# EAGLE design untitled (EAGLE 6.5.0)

## Sheet 1 of 3: NAP a SERVO
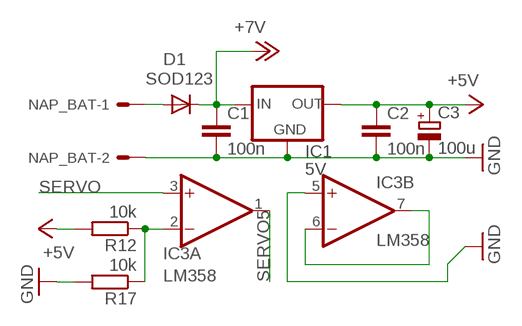
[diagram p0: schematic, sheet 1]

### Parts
C1  100n  C-EUC0805K  [C0805K]
C2  100n  C-EUC0805K  [C0805K]
C3  100u  CPOL-EUE2-5  [E2-5]
D1  SOD123  CGRM4001-G  [SOD-123_MINI-SMA]
IC1  5V  78XXL  [78XXL]
IC3  LM358  TL072D  [SO08]
NAP_BAT  22-27-2021-02  [6410-02]
R12  10k  R-EU_0207/10  [0207/10]
R17  10k  R-EU_0207/10  [0207/10]

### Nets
+7V: C1.1 D1.C IC1.IN ; also sheet 2
GND: C1.2 C2.2 C3.- IC1.GND IC3.5(B:+IN) NAP_BAT.2 R17.2 ; also sheet 2,3
N$2: D1.A NAP_BAT.1
N$6: IC3.6(B:-IN) IC3.7(B:OUT)
N$14: IC3.2(A:-IN) R12.1 R17.1
SERVO: IC3.3(A:+IN) ; also sheet 2
SERVO5: IC3.1(A:OUT) ; also sheet 2
VCC: C2.1 C3.+ IC1.OUT R12.2 ; supply symbol labelled +5V ; also sheet 2,3

## Sheet 2 of 3: HEADER_IO
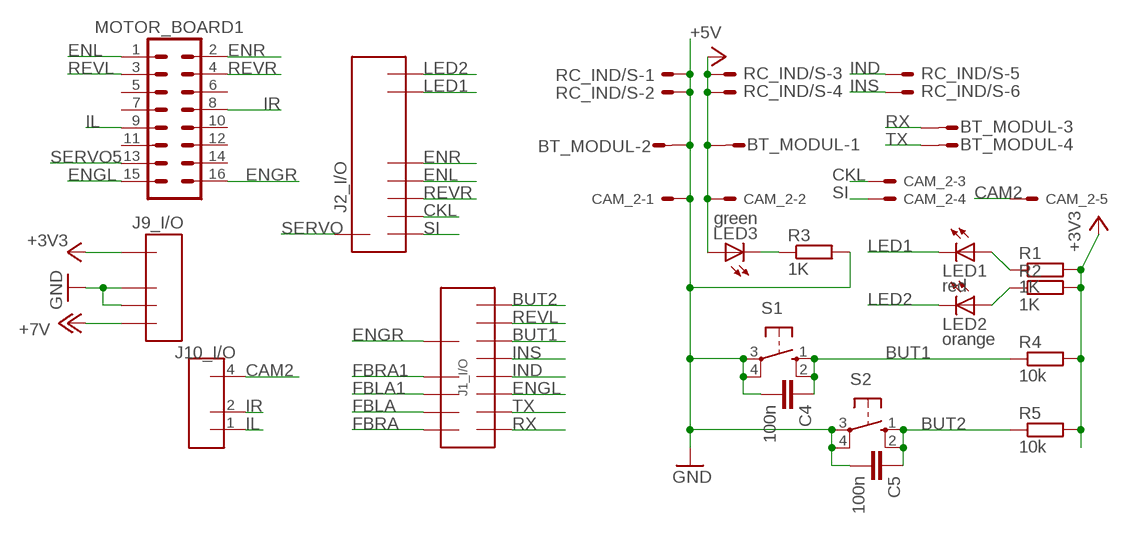
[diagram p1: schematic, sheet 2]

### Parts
BT_MODUL  M04S  [04P]
C4  100n  C-EUC0805K  [C0805K]
C5  100n  C-EUC0805K  [C0805K]
CAM_2  22-27-2051-05  [6410-05]
J1_I/O  DOLNE  [DOLNE]
J2_I/O  HORNE  [HORNE]
J9_I/O  NAP  [NAP]
J10_I/O  ANALOG  [ANALOG]
LED1  red  LED3MM  [LED3MM]
LED2  orange  LED3MM  [LED3MM]
LED3  green  LED3MM  [LED3MM]
MOTOR_BOARD1  ML16  [ML16]
R1  1K  R-EU_R0805  [R0805]
R2  1K  R-EU_R0805  [R0805]
R3  1K  R-EU_R0603  [R0603]
R4  10k  R-EU_R0805  [R0805]
R5  10k  R-EU_R0805  [R0805]
RC_IND/S  ML6E  [ML6]
S1  10-XX  [B3F-10XX]
S2  10-XX  [B3F-10XX]

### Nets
+3V3: J9_I/O.1 R1.2 R2.2 R4.2 R5.2
+7V: J9_I/O.4 ; also sheet 1
BUT1: C4.1 J1_I/O.P$12 R4.1 S1.1(S) S1.2(S1)
BUT2: C5.1 J1_I/O.P$16 R5.1 S2.1(S) S2.2(S1)
CAM2: CAM_2.5 J10_I/O.4
CKL: CAM_2.3 J2_I/O.P$3
ENGL: J1_I/O.P$6 MOTOR_BOARD1.15
ENGR: J1_I/O.P$11 MOTOR_BOARD1.16
ENL: J2_I/O.P$5 MOTOR_BOARD1.1
ENR: J2_I/O.P$6 MOTOR_BOARD1.2
FBLA: J1_I/O.P$3 ; also sheet 3
FBLA1: J1_I/O.P$5 ; also sheet 3
FBRA: J1_I/O.P$1 ; also sheet 3
FBRA1: J1_I/O.P$7 ; also sheet 3
GND: BT_MODUL.2 C4.2 C5.2 CAM_2.1 J9_I/O.2 J9_I/O.3 R3.2 RC_IND/S.1 RC_IND/S.2 S1.3(P) S1.4(P1) S2.3(P) S2.4(P1) ; also sheet 1,3
IL: J10_I/O.1 MOTOR_BOARD1.9
IND: J1_I/O.P$8 RC_IND/S.5
INS: J1_I/O.P$10 RC_IND/S.6
IR: J10_I/O.2 MOTOR_BOARD1.8
LED1: J2_I/O.P$7 LED1.K(C)
LED2: J2_I/O.P$8 LED2.K(C)
N$1: LED1.A R1.1
N$7: LED3.K(C) R3.1
N$15: LED2.A R2.1
REVL: J1_I/O.P$14 MOTOR_BOARD1.3
REVR: J2_I/O.P$4 MOTOR_BOARD1.4
RX: BT_MODUL.3 J1_I/O.P$2
SERVO: J2_I/O.P$1 ; also sheet 1
SERVO5: MOTOR_BOARD1.13 ; also sheet 1
SI: CAM_2.4 J2_I/O.P$2
TX: BT_MODUL.4 J1_I/O.P$4
VCC: BT_MODUL.1 CAM_2.2 LED3.A RC_IND/S.3 RC_IND/S.4 ; supply symbol labelled +5V ; also sheet 1,3
Unconnected: MOTOR_BOARD1.5 MOTOR_BOARD1.6 MOTOR_BOARD1.7 MOTOR_BOARD1.10 MOTOR_BOARD1.11 MOTOR_BOARD1.12 MOTOR_BOARD1.14

## Sheet 3 of 3: CNY70
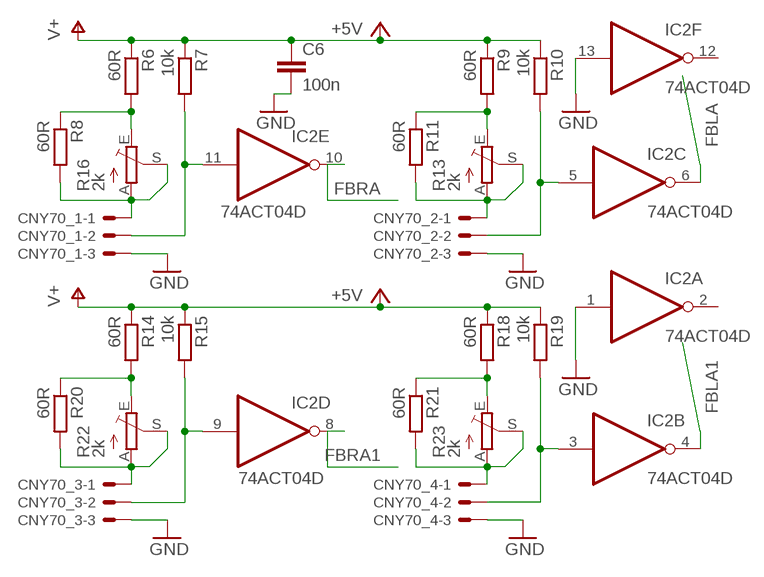
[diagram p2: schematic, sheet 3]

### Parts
C6  100n  C-EUC0805K  [C0805K]
CNY70_1  22-27-2031-03  [6410-03]
CNY70_2  22-27-2031-03  [6410-03]
CNY70_3  22-27-2031-03  [6410-03]
CNY70_4  22-27-2031-03  [6410-03]
IC2  74ACT04D  [SO14]
R6  60R  R-EU_R0603  [R0603]
R7  10k  R-EU_R0603  [R0603]
R8  60R  R-EU_R0603  [R0603]
R9  60R  R-EU_R0603  [R0603]
R10  10k  R-EU_R0603  [R0603]
R11  60R  R-EU_R0603  [R0603]
R13  2k  TRIM_EU-CA6V  [CA6V]
R14  60R  R-EU_R0603  [R0603]
R15  10k  R-EU_R0603  [R0603]
R16  2k  TRIM_EU-CA6V  [CA6V]
R18  60R  R-EU_R0603  [R0603]
R19  10k  R-EU_R0603  [R0603]
R20  60R  R-EU_R0603  [R0603]
R21  60R  R-EU_R0603  [R0603]
R22  2k  TRIM_EU-CA9V  [CA9V]
R23  2k  TRIM_EU-CA9V  [CA9V]

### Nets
FBLA: IC2.6(C:O) ; also sheet 2
FBLA1: IC2.4(B:O) ; also sheet 2
FBRA: IC2.10(E:O) ; also sheet 2
FBRA1: IC2.8(D:O) ; also sheet 2
GND: C6.2 CNY70_1.3 CNY70_2.3 CNY70_3.3 CNY70_4.3 IC2.1(A:I) IC2.13(F:I) ; also sheet 1,2
N$3: R9.2 R11.1 R13.E
N$4: R6.2 R8.1 R16.E
N$5: CNY70_2.1 R11.2 R13.A R13.S
N$8: CNY70_1.1 R8.2 R16.A R16.S
N$9: CNY70_1.2 IC2.11(E:I) R7.2
N$10: CNY70_2.2 IC2.5(C:I) R10.2
N$11: R14.2 R20.1 R22.E
N$12: CNY70_3.1 R20.2 R22.A R22.S
N$13: CNY70_3.2 IC2.9(D:I) R15.2
N$17: CNY70_4.1 R21.2 R23.A R23.S
N$18: CNY70_4.2 IC2.3(B:I) R19.2
N$19: R18.2 R21.1 R23.E
VCC: C6.1 R6.1 R7.1 R9.1 R10.1 R14.1 R15.1 R18.1 R19.1 ; supply symbol labelled V+, +5V ; also sheet 1,2
Unconnected: IC2.2(A:O) IC2.12(F:O)

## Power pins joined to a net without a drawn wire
GND: IC2.7(P:GND) IC3.4(P:V-)
VCC: IC2.14(P:VCC) IC3.8(P:V+)

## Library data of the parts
BT_MODUL = con-amp-quick:M04S: AMP QUICK CONNECTOR; OC_FARNELL: unknown; OC_NEWARK: unknown
C1 C2 C4-C6 = rcl:C-EU: CAPACITOR, European symbol
C3 = rcl:CPOL-EU: POLARIZED CAPACITOR, European symbol
CAM_2 = con-molex:22-?-05: CONNECTOR wire to board 2.54 mm (.1 inch) pitch header; OC_FARNELL: unknown; OC_NEWARK: unknown
CNY70_1-CNY70_4 = con-molex:22-?-03: CONNECTOR wire to board 2.54 mm (.1 inch) pitch header; OC_FARNELL: unknown; OC_NEWARK: unknown
D1 = diode:CGRM400*-G: Molded plasitc,JEDEC SOD-123/Mini SMA
IC1 = v-reg:78XXL: VOLTAGE REGULATOR
IC2 = 74xx-eu:74*04: Hex INVERTER
IC3 = linear:TL072: OP AMP
J1_I/O = con-tfc:DOLNE
J2_I/O = con-tfc:HORNE
J9_I/O = con-tfc:NAP
J10_I/O = con-tfc:ANALOG
LED1-LED3 = led:LED: LED
MOTOR_BOARD1 = con-ml:ML16: HARTING; OC_FARNELL: unknown; OC_NEWARK: unknown
NAP_BAT = con-molex:22-?-02: CONNECTOR; OC_FARNELL: unknown; OC_NEWARK: unknown
R1-R12 R14 R15 R17-R21 = rcl:R-EU_: RESISTOR, European symbol
R13 R16 R22 R23 = pot:TRIM_EU-: POTENTIOMETER
RC_IND/S = con-ml:ML6E: HARTING; OC_FARNELL: unknown; OC_NEWARK: unknown
S1 S2 = switch-omron:10-XX: OMRON SWITCH; MPN: B3F-1000; OC_FARNELL: 176432; OC_NEWARK: 36M3542

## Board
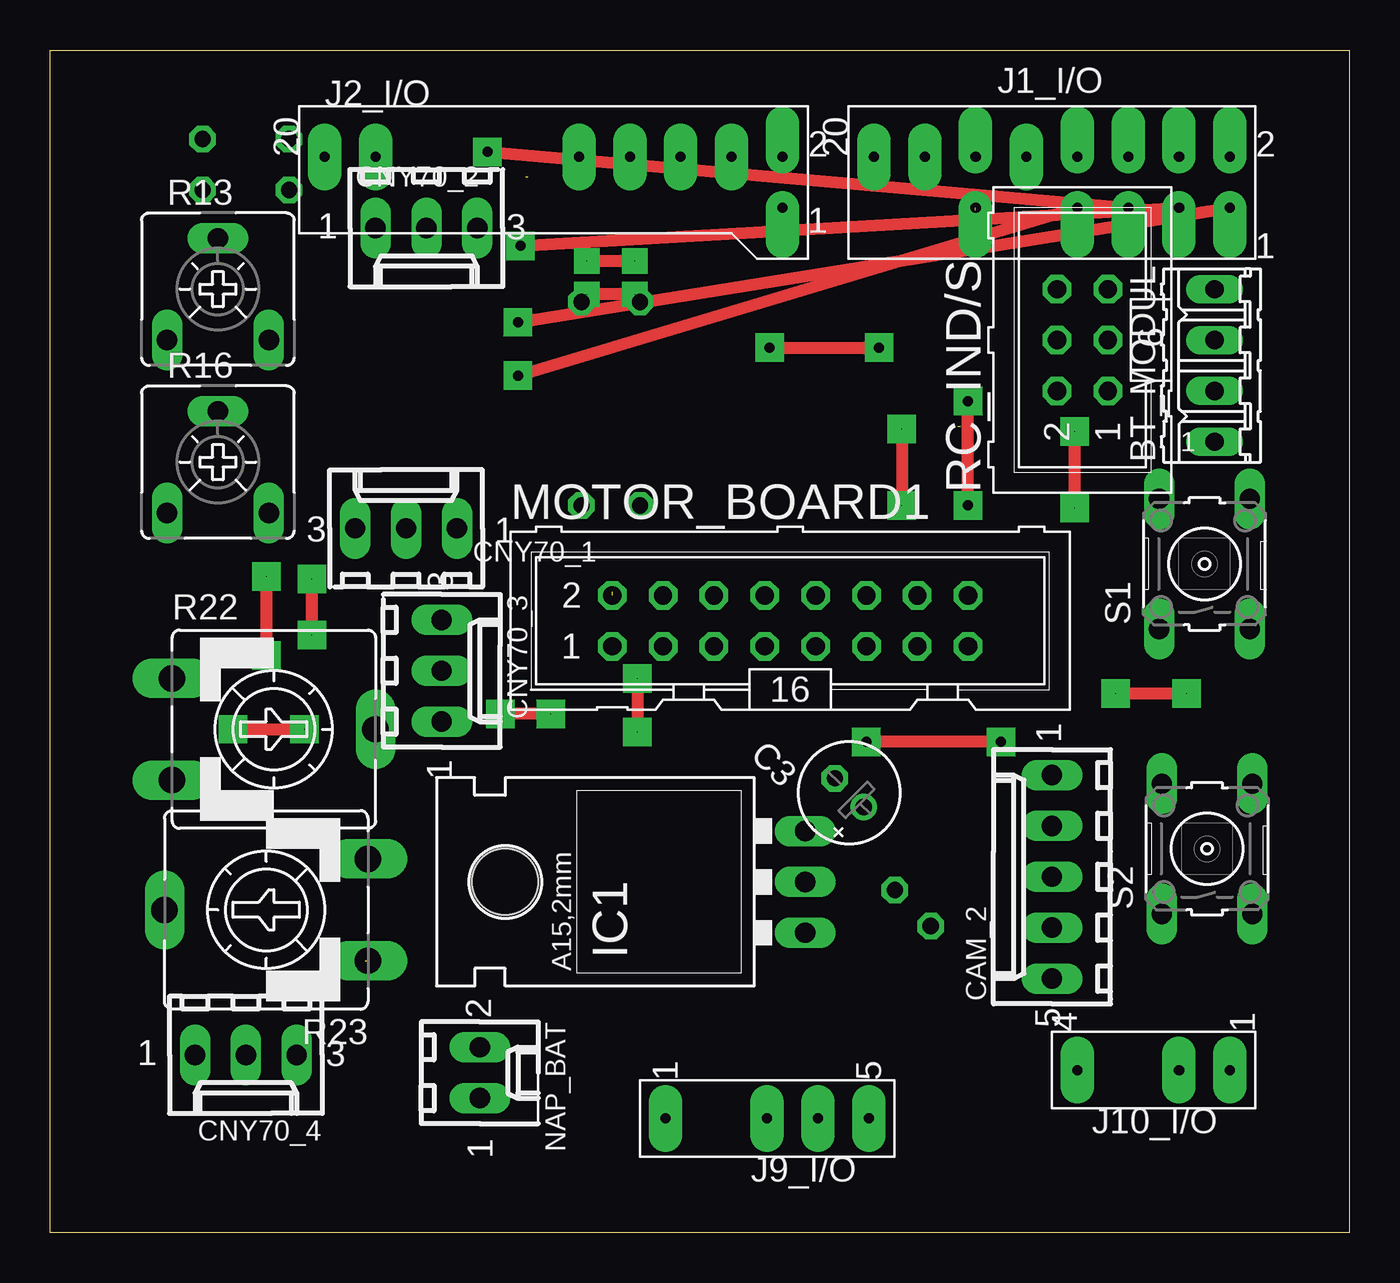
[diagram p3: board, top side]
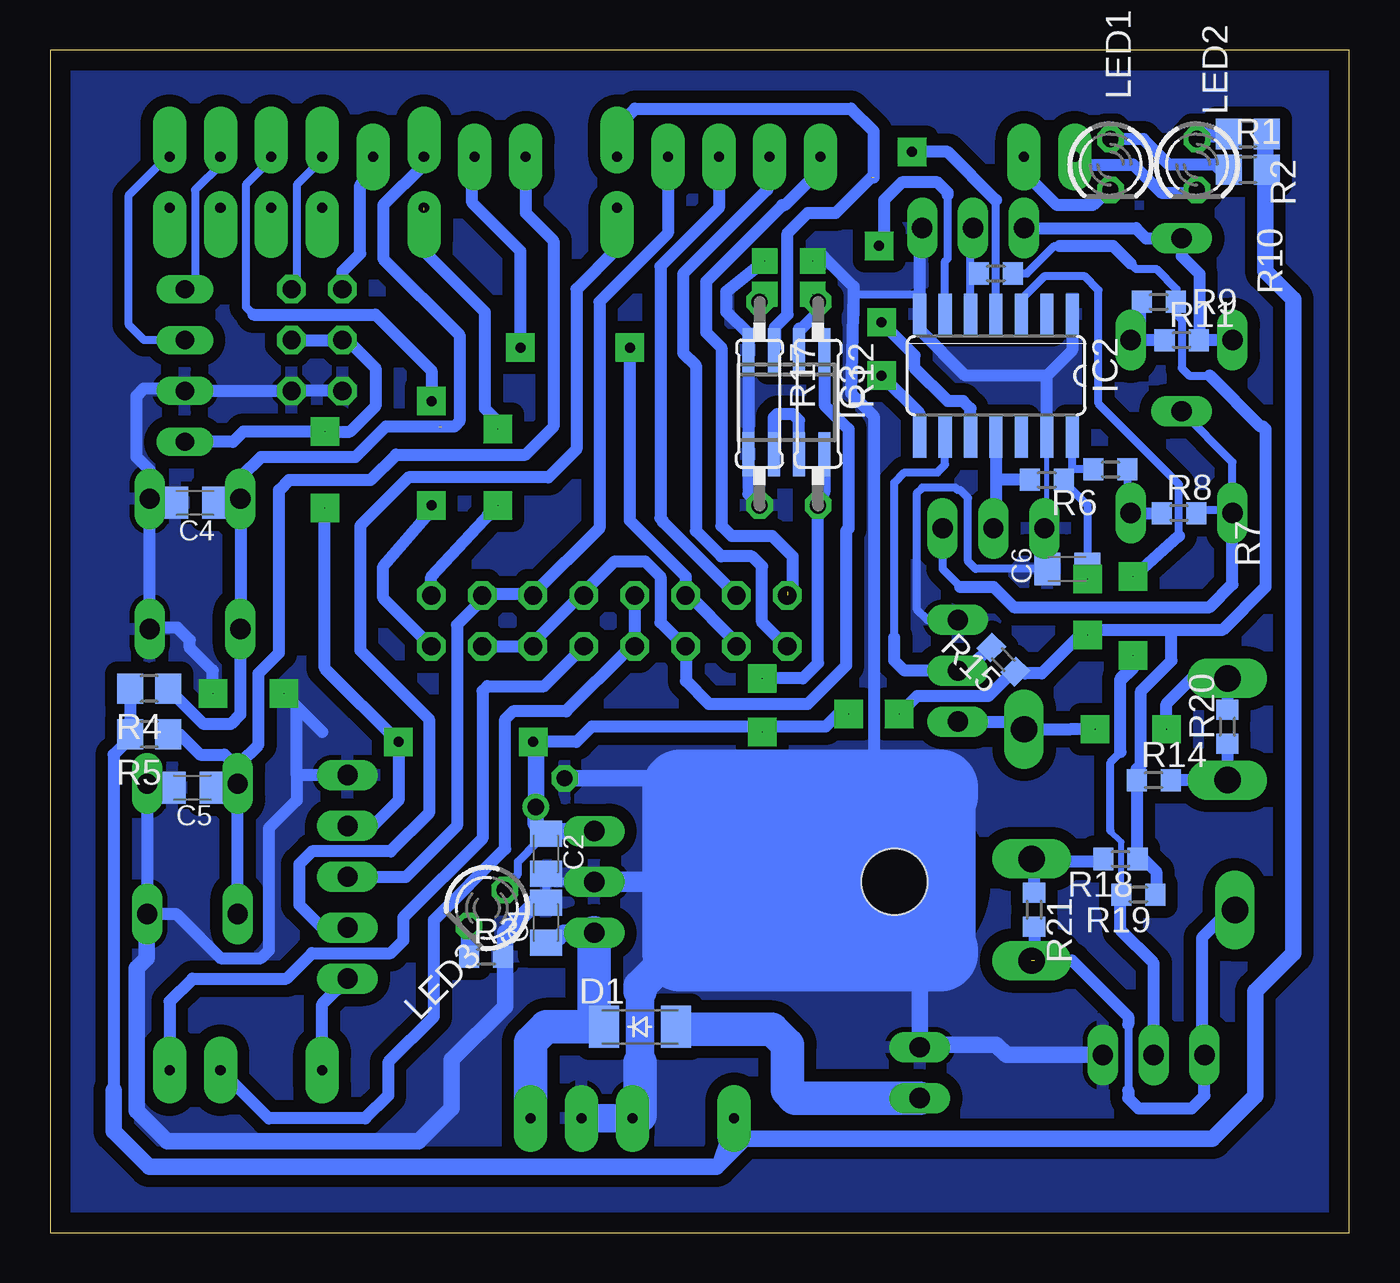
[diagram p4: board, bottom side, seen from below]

Size 64.9 x 59.05 mm. Coordinates in mm from the lower left corner, seen from the top.
Outline: 0,59.05 64.9,59.05 64.9,0 0,0 0,59.05
Copper layers (1*16): Top 0.035mm / dielectric 1.5mm / Bottom 0.035mm
Design rules: minimum track width 10mil, minimum drill 24mil, track to track 8mil, track to pad 8mil, pad to pad 8mil, via to via 8mil, smd to smd 8mil, copper to edge 40mil, drill to drill 8mil, minimum pad ring 10mil, minimum via ring 8mil, stop-mask expansion 4mil, vias tented up to drill 0mil, thermal gap 10mil

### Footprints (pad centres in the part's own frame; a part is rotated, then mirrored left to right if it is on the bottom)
04P = drill 0.914 long: 1 -3.81,0; 2 -1.27,0; 3 1.27,0; 4 3.81,0
C0805K = smd 1.3 x 1.6: 1 -1,0; 2 1,0
E2-5 = drill 0.813 pad 1.27: + -1.016,0 | drill 0.813 pad 1.27 octagon: - 1.016,0
6410-05 = drill 1.016 long: 1 5.08,0; 2 2.54,0; 3 0,0; 4 -2.54,0; 5 -5.08,0
6410-03 = drill 1.016 long: 1 2.54,0; 2 0,0; 3 -2.54,0
SOD-123_MINI-SMA = smd 1.5 x 2.1: A 1.8,0; C -1.8,0
78XXL = drill 1.016 long: GND 0,-3.81; IN -2.54,-3.81; OUT 2.54,-3.81 | hole 3.302: 0,11.176
SO14 = smd 0.66 x 2.032: 1 -3.81,-3.073; 2 -2.54,-3.073; 3 -1.27,-3.073; 4 0,-3.073; 5 1.27,-3.073; 6 2.54,-3.073; 7 3.81,-3.073; 8 3.81,3.073; 9 2.54,3.073; 10 1.27,3.073; 11 0,3.073; 12 -1.27,3.073; 13 -2.54,3.073; 14 -3.81,3.073
SO08 = smd 0.6 x 2.2: 1 -1.905,-2.6; 2 -0.635,-2.6; 3 0.635,-2.6; 4 1.905,-2.6; 5 1.905,2.6; 6 0.635,2.6; 7 -0.635,2.6; 8 -1.905,2.6
DOLNE = drill 0.5 pad 1.676 offset: P$1 8.89,-1.27; P$2 8.89,1.27; P$3 6.35,-1.27; P$4 6.35,1.27; P$5 3.81,-1.27; P$6 3.81,1.27; P$7 1.27,-1.27; P$8 1.27,1.27; P$11 -3.81,-1.27; P$12 -3.81,1.27 | drill 0.5 pad 1.676 long: P$10 -1.27,1.27; P$14 -6.35,1.27; P$16 -8.89,1.27
HORNE = drill 0.5 pad 1.676 offset: P$1 8.89,1.27; P$2 8.89,-1.27 | drill 0.5 pad 1.676 long: P$3 6.35,1.27; P$4 3.81,1.27; P$5 1.27,1.27; P$6 -1.27,1.27; P$7 -11.43,1.27; P$8 -13.97,1.27
NAP = drill 0.5 pad 1.676 long: 1 0,5.08; 2 0,0; 3 0,-2.54; 4 0,-5.08
ANALOG = drill 0.5 pad 1.676 long: 1 0,-3.81; 2 0,-1.27; 4 0,3.81
LED3MM = drill 0.813 octagon: A -1.27,0; K 1.27,0
ML16 = drill 0.914 octagon: 1 -8.89,-1.27; 2 -8.89,1.27; 3 -6.35,-1.27; 4 -6.35,1.27; 5 -3.81,-1.27; 6 -3.81,1.27; 7 -1.27,-1.27; 8 -1.27,1.27; 9 1.27,-1.27; 10 1.27,1.27; 11 3.81,-1.27; 12 3.81,1.27; 13 6.35,-1.27; 14 6.35,1.27; 15 8.89,-1.27; 16 8.89,1.27
6410-02 = drill 1.016 long: 1 1.27,0; 2 -1.27,0
R0805 = smd 1.3 x 1.5: 1 -0.95,0; 2 0.95,0
R0603 = smd 1 x 1.1: 1 -0.85,0; 2 0.85,0
0207/10 = drill 0.813 octagon: 1 -5.08,0; 2 5.08,0
CA6V = drill 1.016 long: A -2.54,-2.54; E 2.54,-2.54; S 0,2.54
CA9V = drill 1.321 long: A -2.54,-5.08; E 2.54,-5.08; S 0,5.08
ML6 = drill 0.914 octagon: 1 -2.54,-1.27; 2 -2.54,1.27; 3 0,-1.27; 4 0,1.27; 5 2.54,-1.27; 6 2.54,1.27
B3F-10XX = drill 1.016 long: 1 -3.251,2.261; 2 3.251,2.261; 3 -3.251,-2.261; 4 3.251,-2.261

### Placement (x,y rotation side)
BT_MODUL  58.17,43.31 90 top
C1  40.13,15.49 90 bottom
C2  40.13,18.92 270 bottom
C3  39.92,21.98 135 top
C4  57.66,36.45 180 bottom
C5  57.78,22.23 180 bottom
C6  14.1,33.15 180 bottom
CAM_2  50.04,17.78 90 top
CNY70_1  17.78,35.18 0 top
CNY70_2  18.8,50.16 180 top
CNY70_3  19.56,28.07 270 top
CNY70_4  9.78,8.89 180 top
D1  35.43,10.29 0 bottom
IC1  33.91,17.53 90 top
IC2  17.65,42.8 180 bottom
IC3  28.12,41.47 180 bottom
J1_I/O  50.04,52.45 0 top
J2_I/O  27.69,52.45 0 top
J9_I/O  35.81,5.71 90 top
J10_I/O  55.12,8.13 90 top
LED1  11.94,53.34 270 bottom
LED2  7.62,53.34 270 bottom
LED3  43.09,16.22 225 bottom
MOTOR_BOARD1  36.97,30.56 0 top
NAP_BAT  21.46,8 270 top
R1  5.08,53.09 0 bottom
R2  5.08,54.86 0 bottom
R3  43.13,13.79 0 bottom
R4  59.94,27.18 180 bottom
R5  59.94,24.89 180 bottom
R6  11.93,38.12 0 bottom
R7  15.11,37.59 180 bottom
R8  8.51,35.94 0 bottom
R9  9.53,46.48 180 bottom
R10  17.65,47.9 180 bottom
R11  8.38,44.58 0 bottom
R12  26.54,41.4 270 bottom
R13  8.38,47.12 0 top
R14  9.78,22.61 0 bottom
R15  17.29,28.62 135 bottom
R16  8.38,38.48 0 top
R17  29.46,41.4 270 bottom
R18  11.43,18.67 180 bottom
R19  10.54,16.89 180 bottom
R20  6.1,25.27 90 bottom
R21  15.75,16.13 270 bottom
R22  11.18,25.15 270 top
R23  10.8,16.13 90 top
RC_IND/S  51.56,44.58 90 top
S1  57.66,33.4 90 top
S2  57.78,19.18 90 top

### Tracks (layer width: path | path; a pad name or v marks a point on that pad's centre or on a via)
+3V3
  Bottom 0.61: 61.72,7.11 61.72,23.88 60.89,24.7 R5.2 R4.2 | 30.73,4.83 30.73,5.46 | 30.73,5.46 30.86,5.46 31.62,3.3 | 30.73,5.46 30.48,5.33 30.23,4.7
  Bottom 0.813: 4.19,52.96 4.19,48.01 2.79,46.61 2.79,13.97 4.7,12.06 4.7,6.86 6.86,4.7 30.23,4.7 31.62,3.3 59.94,3.3 61.72,5.08 61.72,7.11 | 4.19,52.96 4.19,54.42 R2.2 | R1.2 4.13,53.02 4.19,52.96
  Bottom 1.676: J9_I/O.1 30.73,4.83
+7V
  Bottom 0.813: D1.C 37.59,10.29 37.72,10.41 | C1.1 40.12,14.49 39.88,14.73 39.5,14.73 39.24,14.99 IC1.IN
  Bottom 1.676: J9_I/O.4 40.89,9.53 40.13,10.29 37.85,10.29 37.72,10.41 IC1.IN
BUT1  (1 unrouted)
  Bottom 0.406: C4.1 55.5,36.45 55.37,36.58
  Bottom 0.61: J1_I/O.P$12 46.23,53.34 48.26,51.31 48.26,48.64 44.45,44.83 44.45,40.51 44.7,40.26 45.34,40.26 | 45.47,40.26 48.13,40.26 49.66,38.73 54.36,38.73 55.37,37.72 55.37,36.68 S1.2 55.5,36.55 55.5,36.45 55.37,36.45 55.37,30.18 S1.1 55.4,25.88 55.88,25.4 57.22,25.4 R4.1
BUT2
  Bottom 0.61: J1_I/O.P$16 41.15,50.93 39.75,49.53 39.75,40.26 41.15,38.86 47.62,38.86 48.89,37.59 52.96,37.59 53.47,37.08 53.47,28.96 54.48,27.94 54.48,24.38 55.42,23.44 55.42,23.11 | C5.1 55.73,22.23 S2.2 | S2.2 S2.1 55.5,15.95 | S2.2 55.42,22.43 55.42,23.11 | R5.1 58.42,24.89 57.4,23.88 56.19,23.88 55.42,23.11
CAM2
  Bottom 0.61: CAM_2.5 51.31,11.43 J10_I/O.4
CKL
  Bottom 0.61: J2_I/O.P$3 34.04,49.91 37.47,46.48 37.47,35.18 40.77,31.88 43.05,31.88 44.58,30.35 44.58,20.32 47.12,17.78 CAM_2.3
ENGL  (via drill 0.5 pad 1.42)
  Top 0.61: v45.85,36.32 v45.85,41.53
  Bottom 0.406: J1_I/O.P$6 53.85,53.59 55.12,52.32 55.12,46.23 54.74,45.85
  Bottom 0.61: 54.74,45.85 48.64,45.85 45.85,43.05 v45.85,41.53 | MOTOR_BOARD1.15 48.26,31.69 48.26,33.27 45.85,36.07 v45.85,36.32
ENGR  (via drill 0.03 pad 1.42)  (1 unrouted)
  Top 0.61: v42.55,40.13 v42.55,36.32
  Bottom 0.61: MOTOR_BOARD1.16 45.86,32.75 v42.55,36.32 42.93,35.94 43.05,35.81 | 46.23,49.02 46.23,49.4 | 46.23,49.4 46.23,51.05 46.1,51.18 | v42.55,40.13 42.67,40.64 43.18,41.15 43.18,45.97 46.1,48.89 46.1,49.28 46.23,49.4
ENL
  Bottom 0.61: MOTOR_BOARD1.1 28.15,29.29 29.34,30.48 29.34,33.27 29.84,33.78 31.37,33.78 32.64,35.05 32.64,43.31 33.27,43.94 33.27,47.88 29.08,52.07 29.08,53.59 J2_I/O.P$5
ENR  (1 unrouted)
  Bottom 0.61: 28.07,32 27.81,32.26 27.81,33.78 28.83,34.8 30.86,34.8 31.37,35.31 31.37,44.2 32.13,44.96 32.13,47.5 28.32,51.31 28.19,51.31 26.42,53.09 J2_I/O.P$6
FBLA  (via drill 0.5 pad 1.42)
  Top 0.61: v23.5,49.28 J1_I/O.P$3
  Bottom 0.406: IC2.6 20.19,48.51 20.07,48.64 20.07,51.82
  Bottom 0.61: 20.07,51.82 20.07,51.94 20.57,52.45 22.35,52.45 23.24,51.56 23.24,49.53 v23.5,49.28
FBLA1  (via drill 0.5 pad 1.42)
  Top 0.61: v21.84,53.97 J1_I/O.P$5
  Bottom 0.406: IC2.4 17.65,51.56
  Bottom 0.61: 17.65,51.56 20.07,53.97 v21.84,53.97
FBRA  (via drill 0.5 pad 1.42)
  Top 0.61: v23.37,45.47 J1_I/O.P$1
  Bottom 0.61: 23.24,45.47 v23.37,45.47 21.72,43.81 21.72,43.18 20.07,41.53 19.3,41.53 18.92,41.15 IC2.10
FBRA1  (via drill 0.5 pad 1.42)
  Top 0.61: J1_I/O.P$7 v23.37,42.8
  Bottom 0.406: IC2.8 21.46,39.75
  Bottom 0.61: 21.46,39.75 21.46,40.89 v23.37,42.8
GND  (via drill 0.03 pad 1.27, 0.03 pad 1.42)
  Top 0.61: v29.21,48.51 v26.8,48.51 | v56.77,26.92 v53.21,26.92
  Bottom 0.254: CNY70_1.3 15.11,35.31 IC2.13 | 59.11,22.43 58.99,22.43
  Bottom 0.406: C4.2 59.72,36.45 S1.4 | S2.4 59.11,22.43 | 24.77,46.86 21.59,46.86 21.46,47.37 | 13.84,45.08 IC2.1 | IC1.GND 39.73,17.53 C2.2 C1.2 40.76,16.49 | CNY70_3.3 21.08,30.61 21.59,31.11 21.59,36.96 21.34,37.21 19.69,37.21 19.56,37.08 19.43,37.08 19.05,36.7 19.05,33.53 18.67,33.15 C6.2 15.11,33.16 15.11,34.42 | 15,34.43 15.11,34.54
  Bottom 0.61: 21.46,50.29 CNY70_2.3 21.46,50.04 21.46,47.37 IC2.7 21.46,45.08 19.18,42.8 15.11,42.8 | R17.2 30.02,36.88 IC3.5 IC3.4 30.02,44.88 31.12,45.97 31.12,46.99 v29.21,48.51 | RC_IND/S.2 RC_IND/S.1 BT_MODUL.2 | S2.4 60.05,16.89 | 60.05,16.89 S2.3 | S2.3 60.05,15.9 60.07,15.88 | 60.17,17.02 60.05,16.89 | 58.99,22.43 C5.2 | 59.72,36.45 59.82,36.45 59.94,36.32 59.94,30.18 59.39,30.18 59.33,30.23 58.55,30.23 57.91,29.59 57.91,29.21 56.77,28.07 v56.77,26.92 | 58.17,42.16 60.2,42.16 60.58,41.78 60.58,38.73 59.92,38.07 S1.4 | 21.97,20.7 27.43,20.7 | 59.84,30.23 S1.3 | J9_I/O.3 35.43,5.84 | 29.91,16.19 29.59,16.51 | 24.77,46.86 24.77,47.24 26.29,48.77 v26.8,48.51 | 24.77,46.86 24.89,41.91 23.75,40.77 23.75,22.73 23.37,22.23 23.37,19.43 24,18.8 | IC2.13 15.11,42.8 | 13.84,45.08 13.84,44.07 15.11,42.8 | 15.11,35.31 15.11,34.54 15.11,34.42 | S2.3 58.6,15.93 56.39,13.72 54.36,13.72 53.98,14.1 53.98,20.19 52.58,21.59 52.58,22.86 | CAM_2.1 52.58,22.86 | 52.58,22.86 52.58,26.29 v53.21,26.92 51.31,25.02 | 24.77,46.86 24.77,45.85
  Bottom 0.813: 22.61,23.37 22.61,20.57 21.84,19.81 22.99,19.81 | 22.99,19.81 26.29,19.81 | 29.84,17.53 25.4,17.53 | 25.4,17.53 25.27,17.53 24,18.8 22.99,19.81 | C3.- 32.6,22.7 30.35,20.45 30.35,18.8 29.84,18.29 | 25.4,17.53 25.4,16.89 21.46,12.95 NAP_BAT.2 21.34,9.4 17.65,9.4 17.15,8.89 CNY70_4.3 | 40.76,16.49 40.76,16.39 42.16,14.99 42.16,13.84 | 42.16,13.84 42.16,11.3 44.83,8.64 44.83,6.22 46.48,4.57 59.06,4.57 60.58,6.1 60.58,13.21 60.07,13.72 60.07,15.9 S2.3 | R3.2 42.22,13.79 42.16,13.84
  Bottom 1.016: IC1.GND 30.48,17.53 29.84,17.53 29.72,17.65
  Bottom 1.422: J9_I/O.2 J9_I/O.3 | 30.61,17.4 30.48,17.53 | 35.43,8.51 35.43,12.06
  Bottom 1.676: 29.84,17.53 29.84,16.26 29.91,16.19 | 35.43,5.84 35.43,8.51 | 35.43,12.06 35.43,12.32 33.4,14.35 33.4,14.73 29.84,18.29 29.84,17.78 29.72,17.65
  Bottom 3.81: 20.96,20.19 20.57,20.19 20.57,14.35 25.27,14.35 25.27,14.48 31.12,14.48 31.12,14.73 22.99,14.73 22.99,17.4 26.92,17.4 26.92,22.23 33.4,22.23 33.4,13.97 20.45,13.97 20.45,14.1 20.57,14.1 20.57,21.84 20.45,21.84 20.45,22.23 33.27,22.23 33.27,21.08
  Bottom 6.452: 29.72,17.65 27.3,17.65 24.26,20.7 21.97,20.7
  pour Bottom (isolate 0.61): -0.25,59.31 65.02,59.31 64.9,0.76 -0.25,0.76
IL
  Bottom 0.61: 38.24,29.07 MOTOR_BOARD1.9 40.22,27.3 43.05,27.3 43.31,27.05 43.31,19.68 47.24,15.75 47.24,14.61 47.88,13.97 51.82,13.97 53.09,12.7 57.78,12.7 58.93,11.56 J10_I/O.1
IND
  Bottom 0.406: J1_I/O.P$8 51.31,53.59 52.58,52.32 52.58,47.37 RC_IND/S.5
INS
  Bottom 0.61: RC_IND/S.6 50.29,48.01 49.4,48.89 49.4,52.32 48.89,52.83 48.89,53.59 J1_I/O.P$10
IR
  Bottom 0.61: MOTOR_BOARD1.8 35.69,29.08 36.07,29.08 39.12,26.04 41.78,26.04 42.16,25.65 42.16,19.18 45.72,15.62 45.72,10.79 48.01,8.51 48.01,6.86 49.15,5.71 53.98,5.71 J10_I/O.2
LED1
  Bottom 0.61: LED1.K 12.07,52.07 12.83,51.31 14.61,51.31 16.26,52.96 J2_I/O.P$7
LED2
  Bottom 0.61: J2_I/O.P$8 13.46,53.72 13.08,53.34 10.8,53.34 9.4,51.94 7.75,51.94 LED2.K
N$1
  Bottom 0.61: R1.1 6.48,53.09 6.73,53.34 9.02,53.34 10.29,54.61 LED1.A
N$2
  Bottom 0.813: 33.51,10.16 D1.A
  Bottom 1.676: NAP_BAT.1 27.69,6.73 28.07,7.11 28.07,9.4 28.83,10.16 33.51,10.16
N$3
  Bottom 0.406: R9.2 10.38,45.12 R13.E
  Bottom 0.61: R13.E R11.1 9.27,44.62
N$4
  Bottom 0.406: R6.2 11.08,36.1 R16.E
  Bottom 0.61: R16.E R8.1 9.3,36
N$5
  Bottom 0.61: R13.A R11.2 7.49,44.62 7.49,47.88 8.38,48.77 R13.S 10.16,49.66 10.67,50.16 CNY70_2.1
N$6
  Bottom 0.61: IC3.7 27.48,40.56 27.81,40.89 28.58,40.89 28.75,40.72 IC3.6
N$7
  Bottom 0.813: R3.1 LED3.K
N$8
  Bottom 0.406: CNY70_1.1 20.32,33.15 19.43,32.26 | 5.84,34.8 R16.A | R16.A 5.84,38.48 R16.S | 7.49,36.11 6.01,36.11 R16.A
  Bottom 0.61: 7.49,36.11 R8.2 | 19.43,32.26 17.78,32.26 16.76,31.24 6.98,31.24 5.84,32.38 5.84,34.8
N$9
  Bottom 0.61: IC2.11 17.65,37.59 | 17.65,37.59 17.65,35.31 CNY70_1.2 | R7.2 17.65,37.59
N$10
  Bottom 0.406: IC2.5 18.92,47.88 | 18.92,47.88 18.92,50.04 CNY70_2.2 | R10.2 18.9,47.9 18.92,47.88
N$11
  Bottom 0.61: R20.1 R22.E R14.2
N$12  (via drill 0.03 pad 1.42)
  Top 0.61: v9.14,25.15 v12.7,25.15
  Bottom 0.61: R20.2 R22.A 7.87,27.69 9.14,26.42 v9.14,25.15 | CNY70_3.1 16.64,25.53 R22.S 13.97,25.15 v12.7,25.15
N$13
  Bottom 0.406: IC2.9 20.19,38.35 20.57,37.97 22.23,37.97 22.73,37.46 22.73,29.72 | CNY70_3.2 21.08,28.07
  Bottom 0.61: R15.2 18.78,28.47 18.8,28.07 CNY70_3.2 | 21.08,28.07 22.23,28.07 22.73,28.57 22.73,29.72
N$14  (via drill 0.03 pad 1.27)
  Top 0.61: v29.21,46.86 v26.8,46.86
  Bottom 0.61: IC3.2 27.48,45.16 27.36,45.16 26.54,45.97 R12.1 26.54,46.99 26.67,47.12 v26.8,46.86 | R17.1 29.46,46.86 29.34,46.86 v29.21,46.86
N$15
  Bottom 0.813: R2.1 7.37,54.86 LED2.A
N$17  (1 unrouted)
  Bottom 0.406: 11.05,10.41 11.05,7.11
  Bottom 0.61: R23.S 5.97,16.13 7.37,14.73 7.37,9.02 CNY70_4.1 7.24,6.86 7.87,6.22 10.54,6.22 11.05,6.73 11.05,7.11 | R21.2 15.75,13.59 13.84,13.59 11.05,10.79 11.05,10.41
N$18  (via drill 0.03 pad 1.42)
  Top 0.61: v10.8,32.77 v10.8,28.83
  Bottom 0.305: R19.2 11.39,19.52 11.94,20.07
  Bottom 0.406: IC2.3 16.38,46.61 15.24,47.75 13.21,47.75 12.53,47.07 12.53,41.4 8.51,37.38 8.51,34.8 | 11.43,24 11.94,23.5 11.94,20.07
  Bottom 0.61: CNY70_4.2 9.78,13.46 11.43,15.11 11.43,16.85 R19.2 | 11.43,24 11.43,27.56 | 11.43,27.56 11.43,27.69 10.8,28.32 v10.8,28.83 10.8,28.19 11.43,27.56 | v10.8,32.77 8.51,34.8
N$19
  Bottom 0.61: R21.1 15.75,18.54 | R18.2 12.79,18.54 15.75,18.54 | 15.75,18.54 R23.E
N$20
  pour Bottom (isolate 0.61): -0.25,59.31 65.02,59.31 64.9,0.76 -0.25,0.76
REVL  (via drill 0.5 pad 1.42)
  Top 0.61: v35.94,44.2 v41.4,44.2
  Bottom 0.61: MOTOR_BOARD1.3 30.62,29.48 33.15,32 33.15,32.77 35.94,35.56 v35.94,44.2 | v41.4,44.2 41.4,49.02 43.81,51.43 43.81,53.59 J1_I/O.P$14
REVR
  Bottom 0.61: J2_I/O.P$4 31.5,51.18 34.42,48.26 34.42,35.69 34.29,35.56 34.29,35.5 MOTOR_BOARD1.4
RX
  Bottom 0.406: BT_MODUL.3 60.2,44.58 60.96,45.34 60.96,51.82 59.06,53.72 J1_I/O.P$2
SERVO  (1 unrouted)
  Bottom 0.61: J2_I/O.P$1 36.58,55.24 35.69,56.13 24.89,56.13 23.75,54.99 23.75,52.7 | IC3.3 28.7,44.12 28.7,45.21 28.07,45.85 28.07,49.91 27.05,50.93 25.65,50.93 23.88,52.7
SERVO5
  Bottom 0.61: MOTOR_BOARD1.13 40.94,29.29 36.7,33.53 35.18,33.53 34.42,32.77 34.42,30.48 33.15,29.21 33.15,27.56 32,26.42 27.05,26.42 25.15,28.32 25.15,35.05 25.02,35.18 25.02,40.13 26.21,41.32 IC3.1
SI
  Bottom 0.61: J2_I/O.P$2 36.58,49.15 38.61,47.12 38.61,39.12 40.01,37.72 46.99,37.72 49.4,35.31 49.4,29.08 45.97,25.65 45.97,20.96 47.88,19.05 51.82,19.05 52.45,18.41 52.45,16.38 51.31,15.24 CAM_2.4
TX
  Bottom 0.406: J1_I/O.P$4 56.39,53.34 57.66,52.07 57.66,47.62 BT_MODUL.4
VCC  (via drill 0.03 pad 1.42, 0.5 pad 1.42)
  Top 0.61: v47.5,24.51 v40.77,24.51 | v51.18,36.19 v51.18,40 | v25.02,25.91 v22.48,25.91 | v29.34,27.69 v29.34,25.02 | v13.08,29.84 v13.08,32.64
  Bottom 0.406: 26.21,37.03 26.21,36.65 R12.2 | R10.1 16.11,47.9 14.73,49.28 14.48,49.28 | LED3.A 42.19,17.24 41.53,17.91 41.53,18.54 40.51,19.56 40.5,19.56 C2.1 | 10.92,48.39 10.67,48.13 9.65,48.13 8.64,47.12 8.64,46.52 R9.1 8.68,45.89 8.38,45.59 8.38,43.18 8,42.8 6.98,42.8 | R6.1 13.83,38.11 13.84,38.1 | 13.84,38.1 IC2.14 | 13.84,38.1 14.26,37.68 R7.1 14.26,37.5 13.08,36.32 13.08,33.53 13.08,33.16 C6.1
  Bottom 0.61: 6.98,42.8 4.45,40.26 4.32,40.26 4.19,40.13 4.19,32.26 6.35,30.1 8.76,30.1 | IC3.8 26.21,37.03 R12.2 | RC_IND/S.3 RC_IND/S.4 50.04,44.58 48.64,43.18 48.64,41.27 49.91,40 v51.18,40 55.25,40 55.75,39.5 BT_MODUL.1 | v51.18,36.19 51.18,28.19 v47.5,24.51 47.5,21.59 48.77,20.32 CAM_2.2 | R12.2 26.54,36.07 | 40.53,24.27 v40.77,24.51 38.61,24.51 37.85,25.27 29.59,25.27 v29.34,25.02 29.08,25.27 26.16,25.27 25.53,25.91 v25.02,25.91 | R12.2 26.54,28.45 27.3,27.69 v29.34,27.69 | 14.48,49.28 11.81,49.28 10.92,48.39 | R19.1 9.65,16.93 9.65,18.03 10.29,18.67 R18.1 10.63,18.72 R14.1 10.63,23.15 10.41,23.37 10.41,27.05 8.89,28.57 8.89,29.97 8.76,30.1 | 8.76,30.1 13.21,30.1 | 13.21,30.1 13.08,29.97 v13.08,29.84 | C6.1 13.08,33.13 v13.08,32.64 13.08,33.53 | 13.21,30.1 15.37,27.94 16.2,27.94 R15.1 16.79,28.04 18.03,26.8 21.59,26.8 v22.48,25.91
  Bottom 0.813: IC1.OUT 39.99,20.07 C2.1 40.13,19.94 40.64,20.45 C3.+ 40.63,24.38 v40.77,24.51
